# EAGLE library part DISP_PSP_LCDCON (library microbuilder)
Sharp LQ043xx/PSP 24-Bit LCD Display UPPER - FPC Connector w/Upper Contacts BOTTOM - FPC Connector w/Bottom Contacts Use the UPPER connector if the LCD connector is on one side of the board and the LCD will be wrapped around the edge onto the other side of the board (which is what normally happens). Use the BOTTOM connector if the LCD and the connector are on the same side of the board (the cable with be folded directly underneath the LCD).
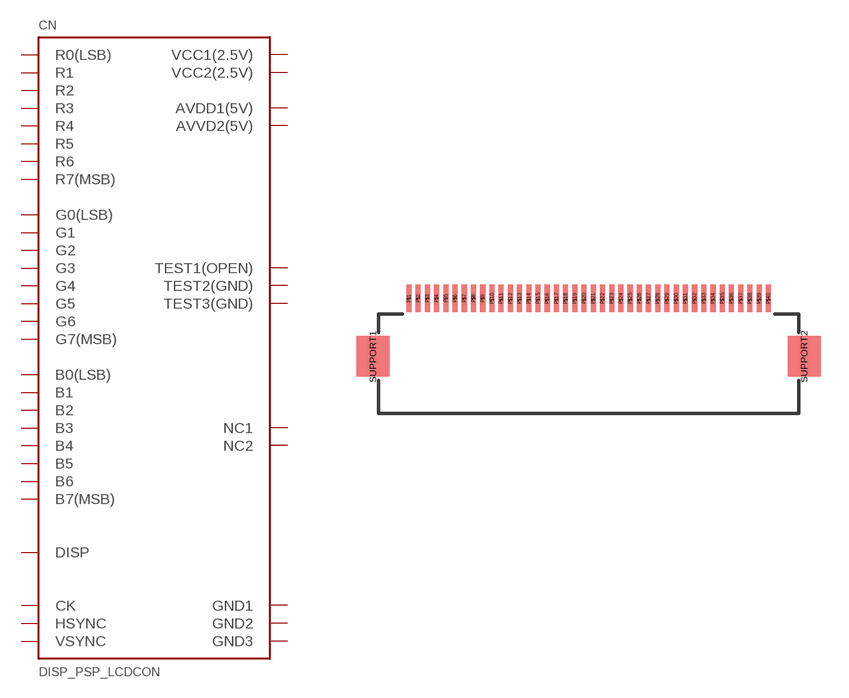
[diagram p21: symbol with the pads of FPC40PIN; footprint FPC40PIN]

Designator prefix CN

## DISP_PSP_LCDCONBOTTOM  [FPC40PIN]
P$1  GND1  pwr
P$2  GND2  pwr
P$3  VCC1(2.5V)  pwr
P$4  VCC2(2.5V)  pwr
P$5  R0(LSB)  in
P$6  R1  in
P$7  R2  in
P$8  R3  in
P$9  R4  in
P$10  R5  in
P$11  R6  in
P$12  R7(MSB)  in
P$13  G0(LSB)  in
P$14  G1  in
P$15  G2  in
P$16  G3  in
P$17  G4  in
P$18  G5  in
P$19  G6  in
P$20  G7(MSB)  in
P$21  B0(LSB)  in
P$22  B1  in
P$23  B2  in
P$24  B3  in
P$25  B4  in
P$26  B5  in
P$27  B6  in
P$28  B7(MSB)  in
P$29  GND3  pwr
P$30  CK
P$31  DISP
P$32  HSYNC
P$33  VSYNC
P$34  NC1  nc
P$35  AVDD1(5V)
P$36  AVVD2(5V)
P$37  NC2  nc
P$38  TEST1(OPEN)
P$39  TEST2(GND)
P$40  TEST3(GND)

## DISP_PSP_LCDCONUPPER  [FPC40PIN]
P$1  TEST3(GND)
P$2  TEST2(GND)
P$3  TEST1(OPEN)
P$4  NC2  nc
P$5  AVVD2(5V)
P$6  AVDD1(5V)
P$7  NC1  nc
P$8  VSYNC
P$9  HSYNC
P$10  DISP
P$11  CK
P$12  GND3  pwr
P$13  B7(MSB)  in
P$14  B6  in
P$15  B5  in
P$16  B4  in
P$17  B3  in
P$18  B2  in
P$19  B1  in
P$20  B0(LSB)  in
P$21  G7(MSB)  in
P$22  G6  in
P$23  G5  in
P$24  G4  in
P$25  G3  in
P$26  G2  in
P$27  G1  in
P$28  G0(LSB)  in
P$29  R7(MSB)  in
P$30  R6  in
P$31  R5  in
P$32  R4  in
P$33  R3  in
P$34  R2  in
P$35  R1  in
P$36  R0(LSB)  in
P$37  VCC2(2.5V)  pwr
P$38  VCC1(2.5V)  pwr
P$39  GND2  pwr
P$40  GND1  pwr

## Footprint FPC40PIN (pad centres in mm)
Sharp LQ043xxx LCD Connector FPC 0.5mm 40 Pin Bottom
smd 0.275 x 1.5: P$1 -9.75,0.75; P$2 -9.25,0.75; P$3 -8.75,0.75; P$4 -8.25,0.75; P$5 -7.75,0.75; P$6 -7.25,0.75; P$7 -6.75,0.75; P$8 -6.25,0.75; P$9 -5.75,0.75; P$10 -5.25,0.75; P$11 -4.75,0.75; P$12 -4.25,0.75; P$13 -3.75,0.75; P$14 -3.25,0.75; P$15 -2.75,0.75; P$16 -2.25,0.75; P$17 -1.75,0.75; P$18 -1.25,0.75; P$19 -0.75,0.75; P$20 -0.25,0.75; P$21 0.25,0.75; P$22 0.75,0.75; P$23 1.25,0.75; P$24 1.75,0.75; P$25 2.25,0.75; P$26 2.75,0.75; P$27 3.25,0.75; P$28 3.75,0.75; P$29 4.25,0.75; P$30 4.75,0.75; P$31 5.25,0.75; P$32 5.75,0.75; P$33 6.25,0.75; P$34 6.75,0.75; P$35 7.25,0.75; P$36 7.75,0.75; P$37 8.25,0.75; P$38 8.75,0.75; P$39 9.25,0.75; P$40 9.75,0.75
smd 1.8 x 2.2: SUPPORT1 -11.7,-2.4; SUPPORT2 11.7,-2.4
